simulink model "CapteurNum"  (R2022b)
settings: Solver=VariableStepAuto  StartTime=0.0  StopTime=10.0  RelTol=1e-3  EnableMultiTasking=on
libraries: simulink x1

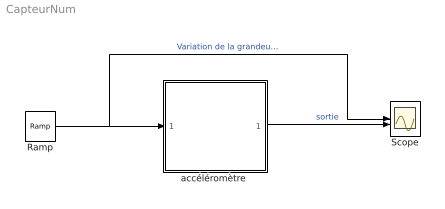
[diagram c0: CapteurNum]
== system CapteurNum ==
  Ramp : simulink/Sources/Ramp  slope=36  start=0  InitialOutput=0
  Scope : Scope  NumInputPorts=2
  "accéléromètre " : Subsystem  mask{pas=36}
      mask prompts: pas "quantification"
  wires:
  Ramp/1 -> Scope/1, "accéléromètre "/1(têta degré)  "Variation de la grandeur d'entrée"
  "accéléromètre "/1(valeur capteur) -> Scope/2  "sortie"

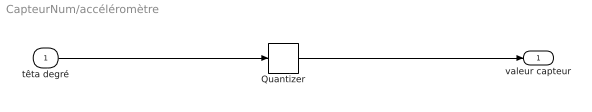
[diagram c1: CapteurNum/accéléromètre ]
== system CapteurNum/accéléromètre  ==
  têta degré : Inport
  Quantizer : Quantizer  QuantizationInterval=pas
  valeur capteur : Outport  VectorParamsAs1DForOutWhenUnconnected=off
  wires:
  têta degré/1 -> Quantizer/1
  Quantizer/1 -> valeur capteur/1
